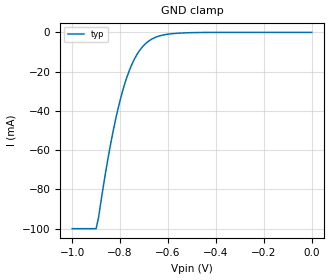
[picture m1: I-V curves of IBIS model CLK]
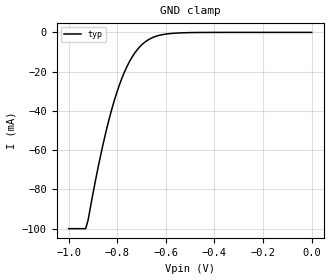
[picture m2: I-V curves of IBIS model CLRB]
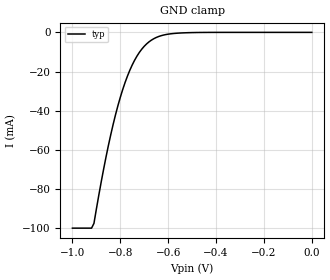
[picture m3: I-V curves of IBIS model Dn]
| Texas Instruments Incorporated
| Marketing part#   Voltage Range   Package-type   #pins/pkg drawing
| TLC59212N   4.5V - 5.5V   PDIP   20-pin N
| TLC59212PW   4.5V - 5.5V   TSSOP   20-pin PW
[IBIS Ver]   4.1
[File name]   tlc59212.ibs
[File Rev]   1.0
[Date]   10/21/2014
[Source]   Model built from lab measurements:
   Texas Instruments Incorporated.
   Analog-eLab, HPA
   12500 TI Blvd
   Dallas, TX -75243
   For Support e-mail: elab_ibis@list.ti.com
[Notes]   Revision History
   Rev 1.0: 10/21/2014
[Disclaimer]  This model is designed as an aid for customers of Texas Instruments
 TI and its licensors and suppliers make no warranties, either expressed
 or implied, with respect to this  model, including the warranties of
 merchantability or fitness for a particular purpose.
 The model is provided solely on an "as is" basis. The entire risk as to
 its quality and performance is with the customer.
[Copyright] (C)Copyright 2014 Texas Instruments Incorporated.
   All rights reserved.
[Component]   TLC59212N
[Manufacturer]  Texas Instruments Incorporated
[Package]   |20-pin PDIP N package
|   typ   min   max
R_pkg   0   0   0
L_pkg   0   0   0
C_pkg   0   0   0
[Pin]   signal_name   model_name   R_pin   L_pin   C_pin
1   CLRB   CLRB   0.22498 10.31934n  1.60197p
2   D1   Dn   0.23474  9.20292n  1.53363p
3   D2   Dn   0.23317  7.75727n  1.10024p
4   D3   Dn   0.21639  6.29691n  0.80586p
5   D4   Dn   0.20651  5.21554n  0.77744p
6   D5   Dn   0.21782  6.64986n  0.91079p
7   D6   Dn   0.22287  7.12520n  1.02702p
8   D7   Dn   0.23800  8.66996n  1.42005p
9   D8   D8   0.23896 10.18340n  1.76261p
10   CLK   CLK   0.23982 11.45174n  1.76438p
11   GND   GND   0.22686 11.27914n  1.75929p
12   Y8B   YnB   0.23528 10.13370n  1.76158p
13   Y7B   YnB   0.23951  8.69076n  1.41907p
14   Y6B   YnB   0.22304  7.12780n  1.02523p
15   Y5B   YnB   0.21495  6.61166n  0.91009p
16   Y4B   YnB   0.20471  5.19044n  0.77855p
17   Y3B   YnB   0.21844  6.32431n  0.80567p
18   Y2B   YnB   0.23601  7.79597n  1.09923p
19   Y1B   YnB   0.23295  9.17852n  1.52964p
20   VCC   POWER   0.22733 10.35074n  1.60186p
[Component]   TLC59212PW
[Manufacturer]  Texas Instruments Incorporated
[Package]   |20-pin TSSOP PW package
|   typ   min   max
R_pkg   0   0   0
L_pkg   0   0   0
C_pkg   0   0   0
[Pin]   signal_name   model_name   R_pin   L_pin   C_pin
1   CLRB   CLRB   0.11593  1.56502n  0.15948p
2   D1   Dn   0.12214  1.67487n  0.17086p
3   D2   Dn   0.11649  1.60341n  0.16299p
4   D3   Dn   0.10229  1.36901n  0.14948p
5   D4   Dn   0.09732  1.28615n  0.13785p
6   D5   Dn   0.09720  1.28430n  0.13882p
7   D6   Dn   0.10211  1.36721n  0.14925p
8   D7   Dn   0.11413  1.57149n  0.16005p
9   D8   D8   0.11919  1.63667n  0.16603p
10   CLK   CLK   0.12307  1.69128n  0.16362p
11   GND   GND   0.11129  1.49094n  0.15604p
12   Y8B   YnB   0.11633  1.58714n  0.16465p
13   Y7B   YnB   0.11551  1.59386n  0.15885p
14   Y6B   YnB   0.10335  1.39264n  0.14869p
15   Y5B   YnB   0.09604  1.27001n  0.13787p
16   Y4B   YnB   0.09736  1.28855n  0.13920p
17   Y3B   YnB   0.10598  1.42935n  0.15123p
18   Y2B   YnB   0.11897  1.64348n  0.16190p
19   Y1B   YnB   0.12078  1.65145n  0.16609p
20   VCC   POWER   0.11863  1.60654n  0.15994p
| Models and submodels in the file (5): CLK (Input), CLRB (Input), Dn (Input), D8 (Input), YnB (Open_drain)
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|   Model CLK
[Model]   CLK
Model_type   Input
Vinl = .8
Vinh = 2
|   typ   min   max
C_comp   3.45p   NA   NA
[Voltage Range]   5   NA   NA
[Temperature Range]   27   NA   NA
[Power Clamp Reference]   5   NA   NA
[GND Clamp Reference]   -0   NA   NA
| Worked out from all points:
|   GND clamp passes 1 mA (typ) near -0.60 V on its own axis
[GND Clamp]
|   Voltage   I(typ)   I(min)   I(max)
-1V       -100mA     NA         NA
-900mV    -100mA     NA         NA
-890mV    -94.48mA   NA         NA
-840mV    -57.27mA   NA         NA
-810mV    -39.65mA   NA         NA
-790mV    -30.11mA   NA         NA
-770mV    -22.29mA   NA         NA
-740mV    -13.55mA   NA         NA
-690mV    -5.34mA    NA         NA
-640mV    -1.966mA   NA         NA
-560mV    -434.7uA   NA         NA
0V        0A         NA         NA
|   Model CLRB
[Model]   CLRB
Model_type   Input
Vinl = .8
Vinh = 2
|   typ   min   max
C_comp   5.5p   NA   NA
[Voltage Range]   5   NA   NA
[Temperature Range]   27   NA   NA
[Power Clamp Reference]   5   NA   NA
[GND Clamp Reference]   -0   NA   NA
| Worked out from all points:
|   GND clamp passes 1 mA (typ) near -0.61 V on its own axis
[GND Clamp]
|   Voltage   I(typ)   I(min)   I(max)
-1V       -100mA     NA         NA
-930mV    -100mA     NA         NA
-920mV    -95.61mA   NA         NA
-890mV    -75.69mA   NA         NA
-860mV    -57.86mA   NA         NA
-810mV    -33.82mA   NA         NA
-780mV    -23.07mA   NA         NA
-750mV    -14.96mA   NA         NA
-690mV    -5.321mA   NA         NA
-640mV    -1.95mA    NA         NA
-560mV    -389.5uA   NA         NA
0V        0A         NA         NA
|   Model Dn
[Model]   Dn
Model_type   Input
Vinl = .8
Vinh = 2
|   typ   min   max
C_comp   5.5p   NA   NA
[Voltage Range]   5   NA   NA
[Temperature Range]   27   NA   NA
[Power Clamp Reference]   5   NA   NA
[GND Clamp Reference]   -0   NA   NA
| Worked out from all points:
|   GND clamp passes 1 mA (typ) near -0.60 V on its own axis
[GND Clamp]
|   Voltage   I(typ)   I(min)   I(max)
-1V       -100mA     NA         NA
-920mV    -100mA     NA         NA
-910mV    -97.55mA   NA         NA
-880mV    -76.57mA   NA         NA
-850mV    -57.95mA   NA         NA
-800mV    -33.2mA    NA         NA
-770mV    -22.31mA   NA         NA
-740mV    -14.19mA   NA         NA
-680mV    -4.841mA   NA         NA
-630mV    -1.722mA   NA         NA
-550mV    -331.1uA   NA         NA
0V        0A         NA         NA
